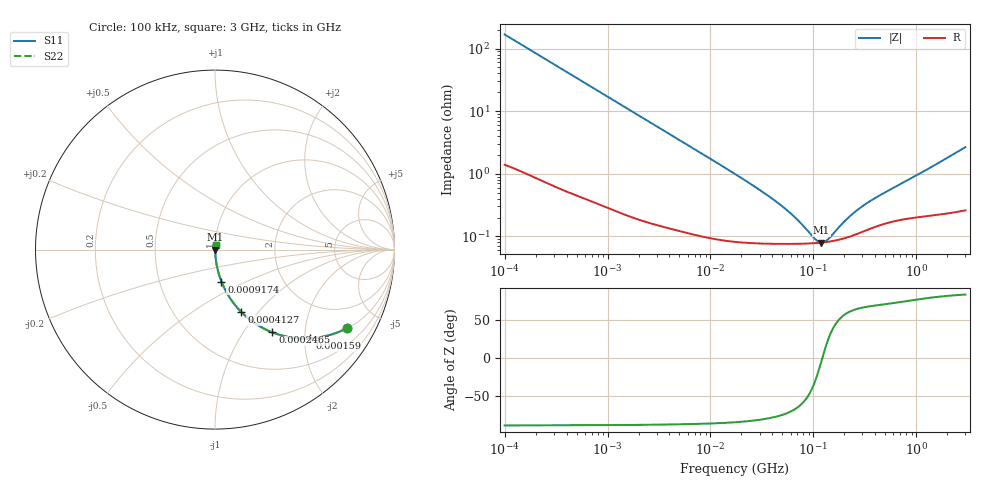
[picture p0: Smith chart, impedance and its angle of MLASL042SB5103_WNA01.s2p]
! MLASL042SB5103_WNA01  S-PARAMETER MODEL  ( Standard Model )
! Model Generated by TAIYO YUDEN Corporation (http://www.ty-top.com)
! Version 1.0
! TAIYO YUDEN Control No. 220601
! Copyright(c) 2009 TAIYO YUDEN CO.,LTD. All Rights Reserved.
! Product Description (link to TY-COMPAS)
! https://ds.yuden.co.jp/TYCOMPAS/or/detail?pn=MLASL042SB5103KWNA01&u=M
! Products Name : Multilayer Ceramic Capacitors
! Characteristics :
!  Capacitance : 0.01 [uF] , Rated Voltage : 10 [V] , TCC : X5R
!  Case Size : 0.4 x 0.2 / 0.016 x 0.008 [mm/inch] , Thickness : 0.2 / 0.008 [mm/inch]
!  (Conditions: Temperature = 25 [degC] , DC Bias Voltage = 0 [V])
! External Node Assignments :
!  1  o---| |---o  2
! GND o---------o GND
! Frequency Range : 100kHz  -  3GHz  [ 401 STEP ]
# MHZ S RI R 50
! Freq[MHz].  S11 Real  S11 Imag  S21 Real  S21 Imag  S12 Real  S12 Imag  S22 Real  S22 Imag
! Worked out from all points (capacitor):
!   401 points, 100 kHz to 3 GHz, reference 50 ohm
!   read as one part in series: C = 9.48 nF near 105.3 kHz
!   lowest |Z| = 79.8 mohm at 119.7 MHz (marker M1)
!   series resonance near 122.1 MHz, so ESL is about 180 pH
!   S11 on the Smith chart (normalised r, x): 100 kHz: 1.03, -3.35; 159 kHz: 1.02, -2.11; 246.5 kHz: 1.01, -1.37; 412.7 kHz: 1.01, -0.82; 917.4 kHz: 1.01, -0.37; 3 GHz: 1.01, +0.05
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0.1  0.7356 -0.4369  0.2644 0.4369  0.2644 0.4369  0.7356 -0.4369
0.159027  0.5272 -0.4945  0.4728 0.4945  0.4728 0.4945  0.5272 -0.4945
0.246461  0.3202 -0.4612  0.6798 0.4612  0.6798 0.4612  0.3202 -0.4612
0.412671  0.1467 -0.3477  0.8533 0.3477  0.8533 0.3477  0.1467 -0.3477
0.562235  0.0864 -0.2741  0.9136 0.2741  0.9136 0.2741  0.0864 -0.2741
0.917447  0.0359 -0.1781  0.9641 0.1781  0.9641 0.1781  0.0359 -0.1781
1.61742  0.0131 -0.104  0.9869 0.104  0.9869 0.104  0.0131 -0.104
3.161081  0.00441 -0.054  0.9956 0.054  0.9956 0.054  0.00441 -0.054
17.7727  0.000905 -0.0096  0.9991 0.0096  0.9991 0.0096  0.000905 -0.0096
32.98988  0.00079 -0.00491  0.9992 0.00491  0.9992 0.00491  0.00079 -0.00491
51.12795  0.000765 -0.00282  0.9992 0.00282  0.9992 0.00282  0.000765 -0.00282
69.65816  0.000763 -0.0017  0.9992 0.0017  0.9992 0.0017  0.000763 -0.0017
97.38194  0.000775 -0.000656  0.9992 0.000656  0.9992 0.000656  0.000775 -0.000656
107.9567  0.000783 -0.000355  0.9992 0.000355  0.9992 0.000355  0.000783 -0.000355
119.6798  0.000795 -5.76e-05  0.9992 5.76e-05  0.9992 5.76e-05  0.000795 -5.76e-05
129.3002  0.000806 0.000164  0.9992 -0.000164  0.9992 -0.000164  0.000806 0.000164
139.694  0.00082 0.000387  0.9992 -0.000387  0.9992 -0.000387  0.00082 0.000387
205.6221  0.000945 0.00154  0.9991 -0.00154  0.9991 -0.00154  0.000945 0.00154
273.0175  0.00112 0.00246  0.9989 -0.00246  0.9989 -0.00246  0.00112 0.00246
371.9668  0.00137 0.00357  0.9986 -0.00357  0.9986 -0.00357  0.00137 0.00357
547.5153  0.00169 0.00521  0.9983 -0.00521  0.9983 -0.00521  0.00169 0.00521
3000  0.00329 0.0263  0.9967 -0.0263  0.9967 -0.0263  0.00329 0.0263
